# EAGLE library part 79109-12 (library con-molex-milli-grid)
RECEPTACAL
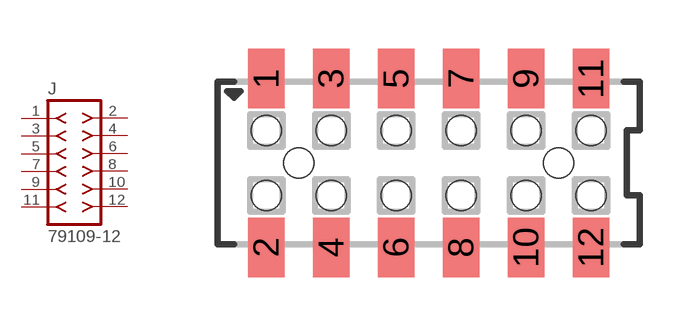
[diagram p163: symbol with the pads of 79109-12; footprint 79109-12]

Designator prefix J

## 79109-12  [79109-12]
1  1  pas
2  2  pas
3  3  pas
4  4  pas
5  5  pas
6  6  pas
7  7  pas
8  8  pas
9  9  pas
10  10  pas
11  11  pas
12  12  pas

## Footprint 79109-12 (pad centres in mm)
RECEPTACAL SMD Dual Row, Vertical, Pass-Thru
smd 1.12 x 1.83: 1 -5,2.6; 2 -5,-2.6; 3 -3,2.6; 4 -3,-2.6; 5 -1,2.6; 6 -1,-2.6; 7 1,2.6; 8 1,-2.6; 9 3,2.6; 10 3,-2.6; 11 5,2.6; 12 5,-2.6
hole 0.914 at -4,0
hole 0.914 at -5,1
hole 0.914 at -5,-1
hole 0.914 at -3,-1
hole 0.914 at -3,1
hole 0.914 at -1,-1
hole 0.914 at -1,1
hole 0.914 at 4,0
hole 0.914 at 1,1
hole 0.914 at 1,-1
hole 0.914 at 3,1
hole 0.914 at 3,-1
hole 0.914 at 5,1
hole 0.914 at 5,-1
